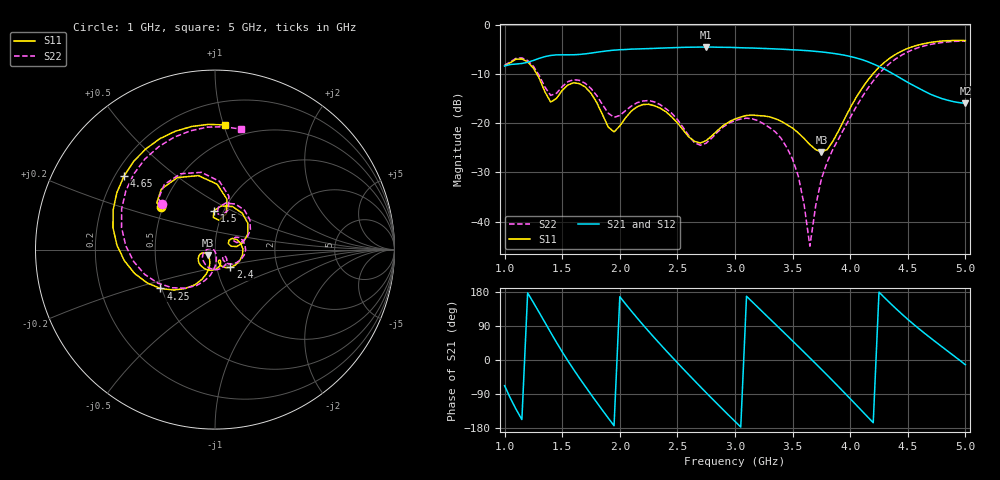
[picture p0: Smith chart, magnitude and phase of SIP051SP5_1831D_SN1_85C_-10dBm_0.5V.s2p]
# GHz  S  dB  R  50
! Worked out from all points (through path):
!   81 points, 1 GHz to 5 GHz, reference 50 ohm
!   highest |S21| = -4.46 dB at 2.75 GHz (marker M1); lowest = -15.9 dB at 5 GHz (marker M2)
!   lowest |S11| = -25.8 dB at 3.75 GHz (marker M3), VSWR 1.11, Z = 46 - j2.79 ohm
!   |S11| at or under -10 dB: 1.28 GHz to 4.195 GHz (2.914 GHz wide, 106 % of centre)
!   |S22| runs from -45.0 to -3.3 dB; largest |S21 - S12| = 0.002
!   S11 on the Smith chart (normalised r, x): 1 GHz: 0.49, +0.27; 1.5 GHz: 0.90, +0.41; 2.4 GHz: 1.16, -0.23; 4.25 GHz: 0.49, -0.25; 4.65 GHz: 0.24, +0.34; 5 GHz: 0.37, +1.01
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1  -8.33 141.9  -8.32 -67.8  -8.32 -67.9  -8.16 139.3
1.2  -7.49 102.6  -7.56 177.0  -7.54 177.1  -7.19 99.9
1.35  -13.59 72.4  -6.41 99.1  -6.39 99.2  -12.61 71.4
1.5  -13.28 91.4  -6.04 21.6  -6.02 21.6  -12.52 85.4
1.7  -12.60 38.8  -5.84 -69.5  -5.84 -69.5  -11.85 40.5
2  -20.53 33.8  -5.01 167.0  -4.99 167.0  -18.40 30.6
2.2  -16.18 1.2  -4.81 93.2  -4.80 93.3  -15.46 9.4
2.35  -16.90 -37.2  -4.68 42.0  -4.67 42.0  -16.18 -20.5
2.4  -17.63 -48.9  -4.63 25.3  -4.62 25.3  -17.00 -30.6
2.55  -21.36 -72.7  -4.52 -23.4  -4.49 -23.3  -20.85 -50.7
2.75  -23.51 -63.9  -4.46 -86.3  -4.45 -86.2  -24.04 -34.6
3  -19.10 -89.2  -4.55 -162.1  -4.55 -162.2  -19.45 -63.0
3.35  -19.06 -146.0  -4.84 94.6  -4.84 94.5  -21.73 -149.0
3.55  -21.95 -164.4  -5.07 35.5  -5.06 35.4  -30.79 170.2
3.65  -24.32 -162.3  -5.23 5.5  -5.24 5.7  -45.03 -132.9
3.7  -25.35 -155.6  -5.35 -9.5  -5.34 -9.5  -36.86 -83.0
3.75  -25.83 -143.7  -5.45 -24.7  -5.45 -24.7  -31.33 -78.1
3.95  -19.14 -108.0  -6.12 -86.4  -6.11 -86.4  -20.94 -89.1
4.25  -8.57 -144.5  -8.42 179.2  -8.39 179.1  -9.91 -138.3
4.35  -6.61 -163.4  -9.62 149.2  -9.64 149.1  -7.64 -160.5
4.65  -3.72 141.1  -13.52 69.5  -13.52 69.4  -4.18 137.0
5  -3.14 85.5  -15.92 -12.6  -15.91 -12.6  -3.27 77.7
